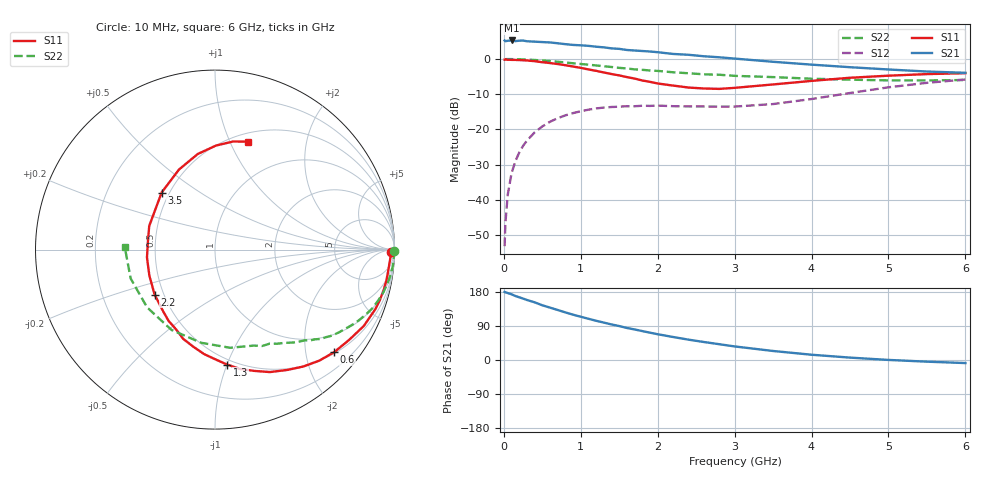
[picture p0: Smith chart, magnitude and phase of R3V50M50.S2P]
! SIEMENS Small Signal Semiconductors
! BFR181
! Si NPN RF Bipolar Junction Transistor in SOT23
! VCE = 0.5 V  IC = 0.5 mA
! Common Emitter S-Parameters:  May  1996
# GHz  S  MA  R  50
!  f  S11  S21  S12  S22
! GHz  MAG  ANG  MAG  ANG  MAG  ANG  MAG  ANG
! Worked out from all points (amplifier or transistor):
!   36 points, 10 MHz to 6 GHz, reference 50 ohm
!   highest |S21| = 5.3 dB at 100 MHz (marker M1)
!   |S21| within 3 dB of that: start of sweep to 1.803 GHz
!   unconditionally stable (mu >= 1): 2.173 GHz to 4.996 GHz; 5.557 GHz to end of sweep
!   at 250 MHz: K = 0.13, MSG = 15.0 dB, |S12| = -24.7 dB
!   at 1.4 GHz: K = 0.67, MSG = 8.3 dB, |S12| = -13.6 dB
!   at 6 GHz: K = 1.01, MAG = 0.2 dB, |S12| = -5.8 dB
!   S11 on the Smith chart (normalised r, x): 10 MHz: 71, -41; 600 MHz: 0.53, -2.60; 1.3 GHz: 0.46, -1.00; 2.2 GHz: 0.45, -0.27; 3.5 GHz: 0.45, +0.36; 6 GHz: 0.59, +1.17
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0.01  0.9791 -0.7  1.832 179.7  0.0022 88.8  0.998 -0.3
0.02  0.9808 -1.4  1.79 178.6  0.0046 89.3  0.9941 -0.8
0.05  0.9772 -3.2  1.815 176.7  0.0117 87.3  0.9985 -1.8
0.1  0.9723 -6.9  1.834 173.4  0.0238 85.8  0.9963 -3.5
0.15  0.9705 -10.1  1.794 168.9  0.0354 82.6  0.9944 -5.5
0.2  0.9664 -13.5  1.821 165.5  0.047 80.2  0.9908 -7.1
0.25  0.9601 -17.2  1.828 162.1  0.0584 77.7  0.9864 -8.9
0.3  0.953 -20.4  1.787 158.4  0.0693 75.5  0.9806 -10.7
0.5  0.9006 -34.0  1.74 144.4  0.1102 66.2  0.9528 -17.3
0.6  0.8761 -40.7  1.718 138.2  0.1285 61.7  0.9354 -20.5
0.8  0.816 -53.0  1.625 125.6  0.1584 53.5  0.8921 -26.3
1.1  0.7108 -72.0  1.537 108.8  0.1908 43.5  0.8304 -33.7
1.3  0.644 -84.0  1.463 98.7  0.2043 37.6  0.7895 -38.1
1.6  0.5535 -102.8  1.343 84.5  0.2137 31.3  0.7345 -43.5
1.8  0.4949 -115.9  1.299 76.3  0.2169 28.6  0.7017 -46.6
2.2  0.4196 -143.3  1.18 60.7  0.2139 24.9  0.6481 -53.3
2.4  0.3932 -158.5  1.148 53.7  0.2122 24.4  0.6275 -56.7
2.8  0.3764 173.1  1.058 41.7  0.2109 25.9  0.598 -63.9
3.5  0.4353 133.1  0.913 23.8  0.2292 33.5  0.5536 -81.2
4.5  0.5415 100.2  0.765 6.3  0.329 37.8  0.509 -118.4
5.5  0.6106 80.5  0.664 -4.4  0.459 27.2  0.4966 -161.1
6  0.6287 73.1  0.637 -8.1  0.5121 19.5  0.503 178.4
